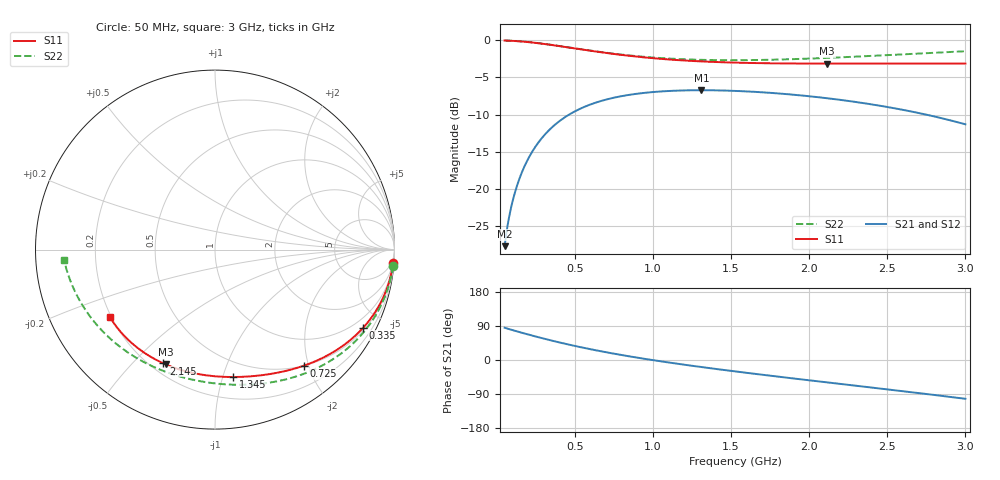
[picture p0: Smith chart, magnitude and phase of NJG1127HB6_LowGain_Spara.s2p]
! Created Mon Dec 09 19:54:13 2013
# hz S ma R 50
! 2 Port Network Data from SP1.SP block
! freq  magS11  angS11  magS21  angS21  magS12  angS12  magS22  angS22
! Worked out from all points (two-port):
!   591 points, 50 MHz to 3 GHz, reference 50 ohm
!   highest |S21| = -6.73 dB at 1.31 GHz (marker M1); lowest = -27.7 dB at 50 MHz (marker M2)
!   |S21| within 3 dB of the highest: 485.8 MHz to 2.686 GHz (2.2 GHz wide, 139 % of centre)
!   lowest |S11| = -3.1 dB at 2.115 GHz (marker M3), VSWR 5.58, Z = 12.7 - j31.5 ohm
!   |S11| at or under -10 dB: nowhere
!   |S22| runs from -2.7 to 0.0 dB; largest |S21 - S12| = 0.002
!   S11 on the Smith chart (normalised r, x): 50 MHz: 2, -26; 335 MHz: 0.59, -3.97; 725 MHz: 0.50, -1.92; 1.345 GHz: 0.37, -1.08; 2.145 GHz: 0.25, -0.62; 3 GHz: 0.19, -0.29
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5e7  0.9944 -4.4  0.04126 85.2  0.04136 85.2  0.9955 -5.2
8e7  0.9919 -7.0  0.06571 81.3  0.06588 81.3  0.9929 -8.2
1e8  0.9895 -8.7  0.08183 78.9  0.08203 78.9  0.9906 -10.3
1.25e8  0.9859 -10.8  0.1017 76.0  0.102 76.0  0.987 -12.8
1.55e8  0.9807 -13.4  0.125 72.5  0.1254 72.5  0.9817 -15.8
2.35e8  0.9625 -20.0  0.1839 63.5  0.1843 63.5  0.9635 -23.7
3.35e8  0.9335 -27.7  0.2487 52.9  0.2493 52.9  0.9345 -32.9
4.35e8  0.9013 -34.9  0.3029 43.1  0.3037 43.1  0.9024 -41.6
5.45e8  0.8658 -42.1  0.3504 33.1  0.3513 33.1  0.8673 -50.3
7.25e8  0.814 -52.7  0.405 18.5  0.406 18.6  0.817 -63.2
8.75e8  0.7794 -60.5  0.4333 7.8  0.4344 7.9  0.7846 -72.8
1.035e9  0.7511 -68.2  0.4511 -2.6  0.4523 -2.5  0.7598 -82.2
1.31e9  0.7198 -80.4  0.461 -18.6  0.4622 -18.5  0.7374 -97.1
1.345e9  0.717 -81.9  0.4608 -20.5  0.4621 -20.4  0.7361 -98.9
1.525e9  0.7063 -89.5  0.4561 -30.1  0.4574 -30.0  0.7334 -108.0
1.775e9  0.6986 -99.7  0.4408 -42.7  0.4421 -42.5  0.7395 -120.2
2.02e9  0.6961 -109.5  0.4178 -54.6  0.4192 -54.4  0.7532 -131.7
2.115e9  0.696 -113.2  0.4072 -59.1  0.4085 -59.0  0.76 -136.1
2.145e9  0.696 -114.4  0.4036 -60.6  0.405 -60.4  0.7623 -137.5
2.51e9  0.6972 -128.5  0.3541 -78.0  0.3554 -77.8  0.7943 -154.1
2.765e9  0.6975 -138.3  0.3132 -90.5  0.3146 -90.2  0.8193 -165.6
3e9  0.6963 -147.1  0.2719 -102.4  0.2732 -102.1  0.8426 -176.0
